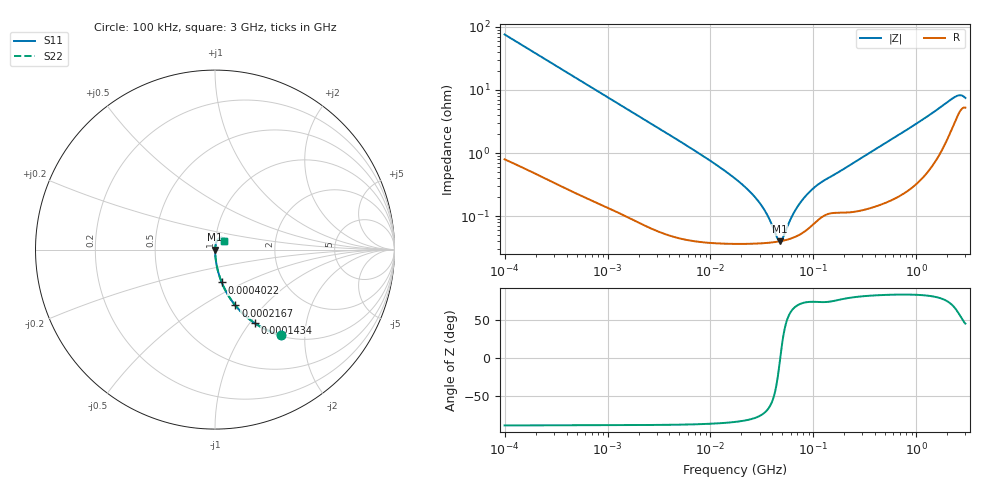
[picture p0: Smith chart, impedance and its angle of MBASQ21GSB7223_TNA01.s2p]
! MBASQ21GSB7223_TNA01  S-PARAMETER MODEL  ( Standard Model )
! Model Generated by TAIYO YUDEN Corporation (http://www.ty-top.com)
! Version 1.0
! TAIYO YUDEN Control No. 220601
! Copyright(c) 2013 TAIYO YUDEN CO.,LTD. All Rights Reserved.
! Product Description (link to TY-COMPAS)
! https://ds.yuden.co.jp/TYCOMPAS/or/detail?pn=MBASQ21GSB7223KTNA01&u=M
! Products Name : Multilayer Ceramic Capacitors
! Characteristics :
!  Capacitance : 0.022 [uF] , Rated Voltage : 250 [V] , TCC : X7R
!  Case Size : 2.0 x 1.25 / 0.079 x 0.049 [mm/inch] , Thickness : 1.25 / 0.049 [mm/inch]
!  (Conditions: Temperature = 25 [degC] , DC Bias Voltage = 0 [V])
! External Node Assignments :
!  1  o---| |---o  2
! GND o---------o GND
! Frequency Range : 100kHz  -  3GHz  [ 401 STEP ]
# MHZ S RI R 50
! Freq[MHz].  S11 Real  S11 Imag  S21 Real  S21 Imag  S12 Real  S12 Imag  S22 Real  S22 Imag
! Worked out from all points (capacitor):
!   401 points, 100 kHz to 3 GHz, reference 50 ohm
!   read as one part in series: C = 20.9 nF near 105.3 kHz
!   lowest |Z| = 39.9 mohm at 47.32 MHz (marker M1)
!   series resonance near 47.65 MHz, so ESL is about 530 pH
!   S11 on the Smith chart (normalised r, x): 100 kHz: 1.02, -1.52; 143.4 kHz: 1.01, -1.06; 216.7 kHz: 1.01, -0.70; 402.2 kHz: 1.01, -0.38; 3 GHz: 1.10, +0.11
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0.1  0.367 -0.4768  0.633 0.4768  0.633 0.4768  0.367 -0.4768
0.14345  0.2223 -0.4101  0.7777 0.4101  0.7777 0.4101  0.2223 -0.4101
0.216663  0.1135 -0.311  0.8865 0.311  0.8865 0.311  0.1135 -0.311
0.402172  0.0375 -0.1831  0.9625 0.1831  0.9625 0.1831  0.0375 -0.1831
0.562235  0.0203 -0.1338  0.9797 0.1338  0.9797 0.1338  0.0203 -0.1338
3.161081  0.00117 -0.0246  0.9988 0.0246  0.9988 0.0246  0.00117 -0.0246
9.574722  0.000439 -0.00786  0.9996 0.00786  0.9996 0.00786  0.000439 -0.00786
17.7727  0.000376 -0.0038  0.9996 0.0038  0.9996 0.0038  0.000376 -0.0038
24.21403  0.000369 -0.00241  0.9996 0.00241  0.9996 0.00241  0.000369 -0.00241
30.53531  0.000371 -0.00152  0.9996 0.00152  0.9996 0.00152  0.000371 -0.00152
36.57227  0.000378 -0.000886  0.9996 0.000886  0.9996 0.000886  0.000378 -0.000886
44.94634  0.000393 -0.000194  0.9996 0.000194  0.9996 0.000194  0.000393 -0.000194
47.32384  0.000398 -2.27e-05  0.9996 2.27e-05  0.9996 2.27e-05  0.000398 -2.27e-05
51.12795  0.000408 0.000234  0.9996 -0.000234  0.9996 -0.000234  0.000408 0.000234
61.23616  0.000444 0.000845  0.9996 -0.000845  0.9996 -0.000845  0.000444 0.000845
69.65816  0.000486 0.0013  0.9995 -0.0013  0.9995 -0.0013  0.000486 0.0013
97.38194  0.00072 0.00256  0.9993 -0.00256  0.9993 -0.00256  0.00072 0.00256
122.8043  0.000991 0.00341  0.999 -0.00341  0.999 -0.00341  0.000991 0.00341
547.5153  0.00196 0.0156  0.998 -0.0156  0.998 -0.0156  0.00196 0.0156
2318.426  0.0324 0.0661  0.9676 -0.0661  0.9676 -0.0661  0.0324 0.0661
2637.286  0.0472 0.0631  0.9528 -0.0631  0.9528 -0.0631  0.0472 0.0631
3000  0.0522 0.048  0.9478 -0.048  0.9478 -0.048  0.0522 0.048
